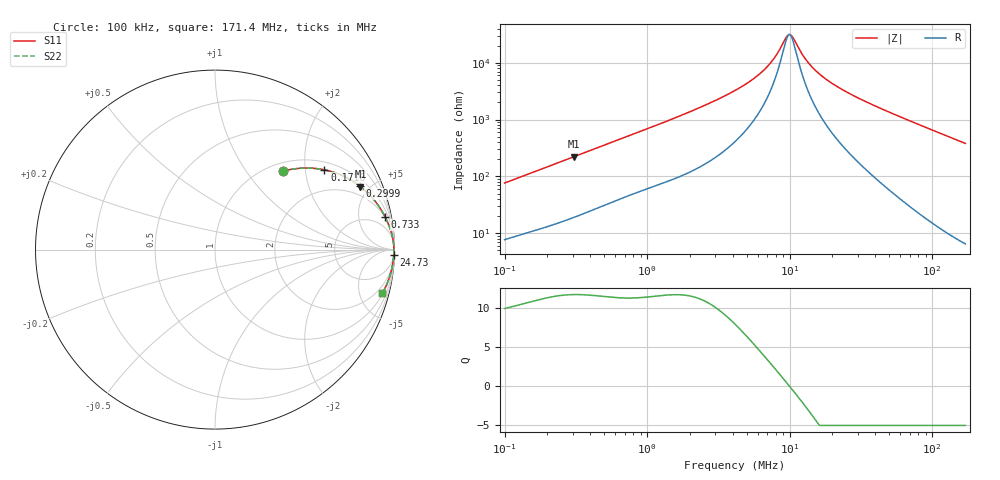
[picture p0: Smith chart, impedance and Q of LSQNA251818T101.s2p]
! LSQNA251818T101  S-PARAMETER MODEL  ( General Type )
! Model Generated by TAIYO YUDEN Corporation (http://www.ty-top.com)
! Version 2.0
! TAIYO YUDEN Control No. 100810NF25SB-FKC
! Copyright(c) 2007 TAIYO YUDEN CO.,LTD. All Rights Reserved.
! Product Description (link to TY-COMPAS)
! https://ds.yuden.co.jp/TYCOMPAS/or/detail?pn=LSQNA251818T101K&u=M
! Products Name : Inductors
! Characteristics :
!  Inductance : 100 uH , SRF(min) : 9.0 MHz , DC Resistance(max) : 2.73 Ohm
!  Rated Current : Saturation :60 mA , Temp Rise : 260 mA (40 degC)
!  Case Size : 2.5 x 1.8 / 0.098 x 0.071 [mm/inch] , Thickness : 1.8 / 0.071 [mm/inch]
!  (Conditions: Temperature = 25 degC , DC Bias Current/Voltage = 0A / 0V)
! External Node Assignments :
!  1  o---GGG---o  2
! GND o---------o GND
! Frequency Range : 0.1MHz  -  171.398534MHz  [ 402 STEP ]
# MHz S RI R 50
! Freq[MHz].  S11 Real  S11 Imag  S21 Real  S21 Imag  S12 Real  S12 Imag  S22 Real  S22 Imag
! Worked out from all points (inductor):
!   401 points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, 100 kHz to 171.4 MHz, reference 50 ohm
!   read as one part in series: L = 119 uH near 103.8 kHz
!   highest Q = 11.6 at 305.6 kHz (marker M1), where L = 115 uH
!   self-resonance near 9.931 MHz
!   S11 on the Smith chart (normalised r, x): 100 kHz: 1.15, +1.52; 171.6 kHz: 1.23, +2.54; 299.9 kHz: 1.37, +4.33; 733 kHz: 2, +10; 24.73 MHz: 7, -62; 171.4 MHz: 1.13, -7.60
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0.1  0.3809 0.4376  0.6191 -0.4376  0.6191 -0.4376  0.3809 0.4376
0.17158  0.6095 0.4444  0.3905 -0.4444  0.3905 -0.4444  0.6095 0.4444
0.299927  0.8055 0.3552  0.1945 -0.3552  0.1945 -0.3552  0.8055 0.3552
0.305563  0.8105 0.3513  0.1895 -0.3513  0.1895 -0.3513  0.8105 0.3513
0.348094  0.8426 0.3238  0.1574 -0.3238  0.1574 -0.3238  0.8426 0.3238
0.732988  0.9478 0.1822  0.0522 -0.1822  0.0522 -0.1822  0.9478 0.1822
1.211692  0.9757 0.1164  0.0243 -0.1164  0.0243 -0.1164  0.9757 0.1164
2.504425  0.9916 0.056  0.00836 -0.056  0.00836 -0.056  0.9916 0.056
4.140031  0.9952 0.0303  0.00478 -0.0303  0.00478 -0.0303  0.9952 0.0303
5.473673  0.9961 0.0194  0.00388 -0.0194  0.00388 -0.0194  0.9961 0.0194
6.843827  0.9965 0.0118  0.00347 -0.0118  0.00347 -0.0118  0.9965 0.0118
7.796401  0.9967 0.00761  0.00332 -0.00761  0.00332 -0.00761  0.9967 0.00761
9.391703  0.9968 0.00186  0.00319 -0.00186  0.00319 -0.00186  0.9968 0.00186
9.931146  0.9968 0.000155  0.00317 -0.000155  0.00317 -0.000155  0.9968 0.000155
10.50158  0.9968 -0.00155  0.00315 0.00155  0.00315 0.00155  0.9968 -0.00155
12.41708  0.9968 -0.00672  0.00316 0.00672  0.00316 0.00672  0.9968 -0.00672
14.41119  0.9968 -0.0115  0.00323 0.0115  0.00323 0.0115  0.9968 -0.0115
18.01855  0.9966 -0.0191  0.00344 0.0191  0.00344 0.0191  0.9966 -0.0191
24.72665  0.9959 -0.0316  0.00407 0.0316  0.00407 0.0316  0.9959 -0.0316
50.16444  0.9914 -0.0733  0.00856 0.0733  0.00856 0.0733  0.9914 -0.0733
94.4684  0.9765 -0.1399  0.0235 0.1399  0.0235 0.1399  0.9765 -0.1399
171.3985  0.9317 -0.2439  0.0683 0.2439  0.0683 0.2439  0.9317 -0.2439
